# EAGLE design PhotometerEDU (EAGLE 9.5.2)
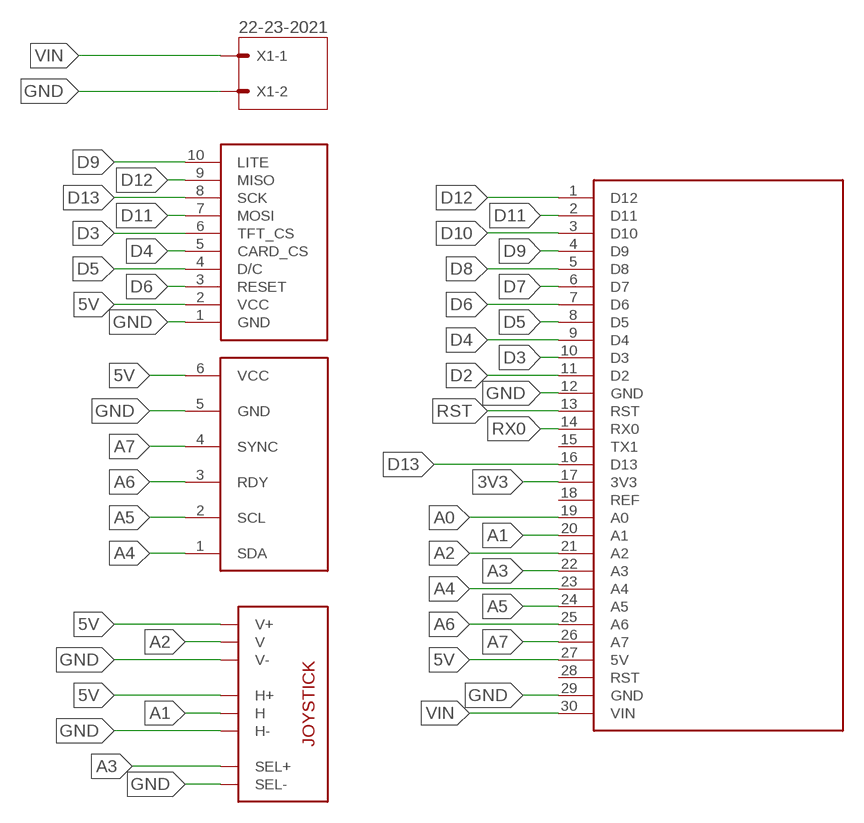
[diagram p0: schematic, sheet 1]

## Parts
78511-406  SAURON  [SAURON]
A000005  NANO  [NANO]
COM-09032  JOYSTICKPTH  [JOYSTICK]
EXP-R15-111  DISPLAY  [DISPLAY]
X1  22-23-2021  [22-23-2021]

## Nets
3V3: A000005.17(3V3)
5V: 78511-406.6(VCC) A000005.27(5V) COM-09032.H1(H+) COM-09032.V1(V+) EXP-R15-111.2(VCC)
A0: A000005.19(A0)
A1: A000005.20(A1) COM-09032.H2(H)
A2: A000005.21(A2) COM-09032.V2(V)
A3: A000005.22(A3) COM-09032.B1A(SEL+)
A4: 78511-406.1(SDA) A000005.23(A4)
A5: 78511-406.2(SCL) A000005.24(A5)
A6: 78511-406.3(RDY) A000005.25(A6)
A7: 78511-406.4(SYNC) A000005.26(A7)
D2: A000005.11(D2)
D3: A000005.10(D3) EXP-R15-111.6(TFT_CS)
D4: A000005.9(D4) EXP-R15-111.5(CARD_CS)
D5: A000005.8(D5) EXP-R15-111.4(D/C)
D6: A000005.7(D6) EXP-R15-111.3(RESET)
D7: A000005.6(D7)
D8: A000005.5(D8)
D9: A000005.4(D9) EXP-R15-111.10(LITE)
D10: A000005.3(D10)
D11: A000005.2(D11) EXP-R15-111.7(MOSI)
D12: A000005.1(D12) EXP-R15-111.9(MISO)
D13: A000005.16(D13) EXP-R15-111.8(SCK)
GND: 78511-406.5(GND) A000005.12(GND) A000005.29(GND) COM-09032.B2A(SEL-) COM-09032.H3(H-) COM-09032.V3(V-) EXP-R15-111.1(GND) X1.2
RST: A000005.13(RST)
RX0: A000005.14(RX0)
VIN: A000005.30(VIN) X1.1
Unconnected: A000005.15(TX1) A000005.18(REF) A000005.28(RST)

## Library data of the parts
78511-406 = Lego:SAURON
A000005 = Lego:NANO
COM-09032 = SparkFun-Electromechanical:JOYSTICK: Thumb Joystick Joystick commonly found in PS2 controllers. Two pots and a select switch. Footprint proven. Spark Fun Electronics SKU : COM-09032
EXP-R15-111 = Lego:DISPLAY
X1 = con-molex:22-23-2021: .100" (2.54mm) Center Header - 2 Pin; MF: MOLEX; MPN: 22-23-2021; OC_FARNELL: 1462926; OC_NEWARK: 25C3832

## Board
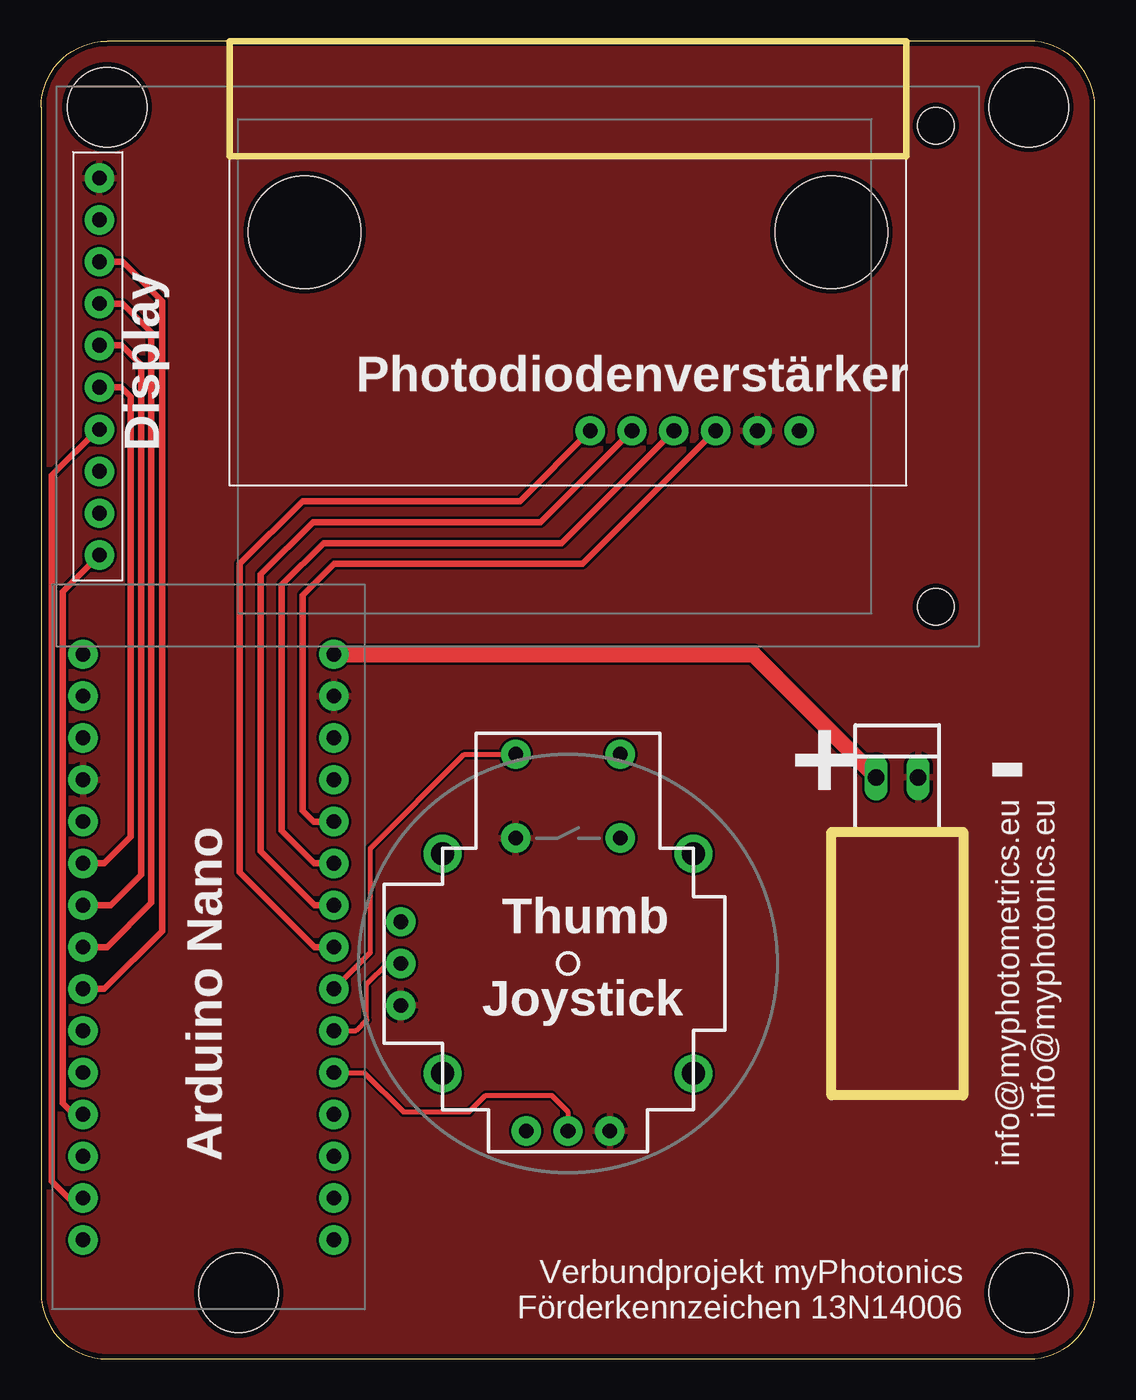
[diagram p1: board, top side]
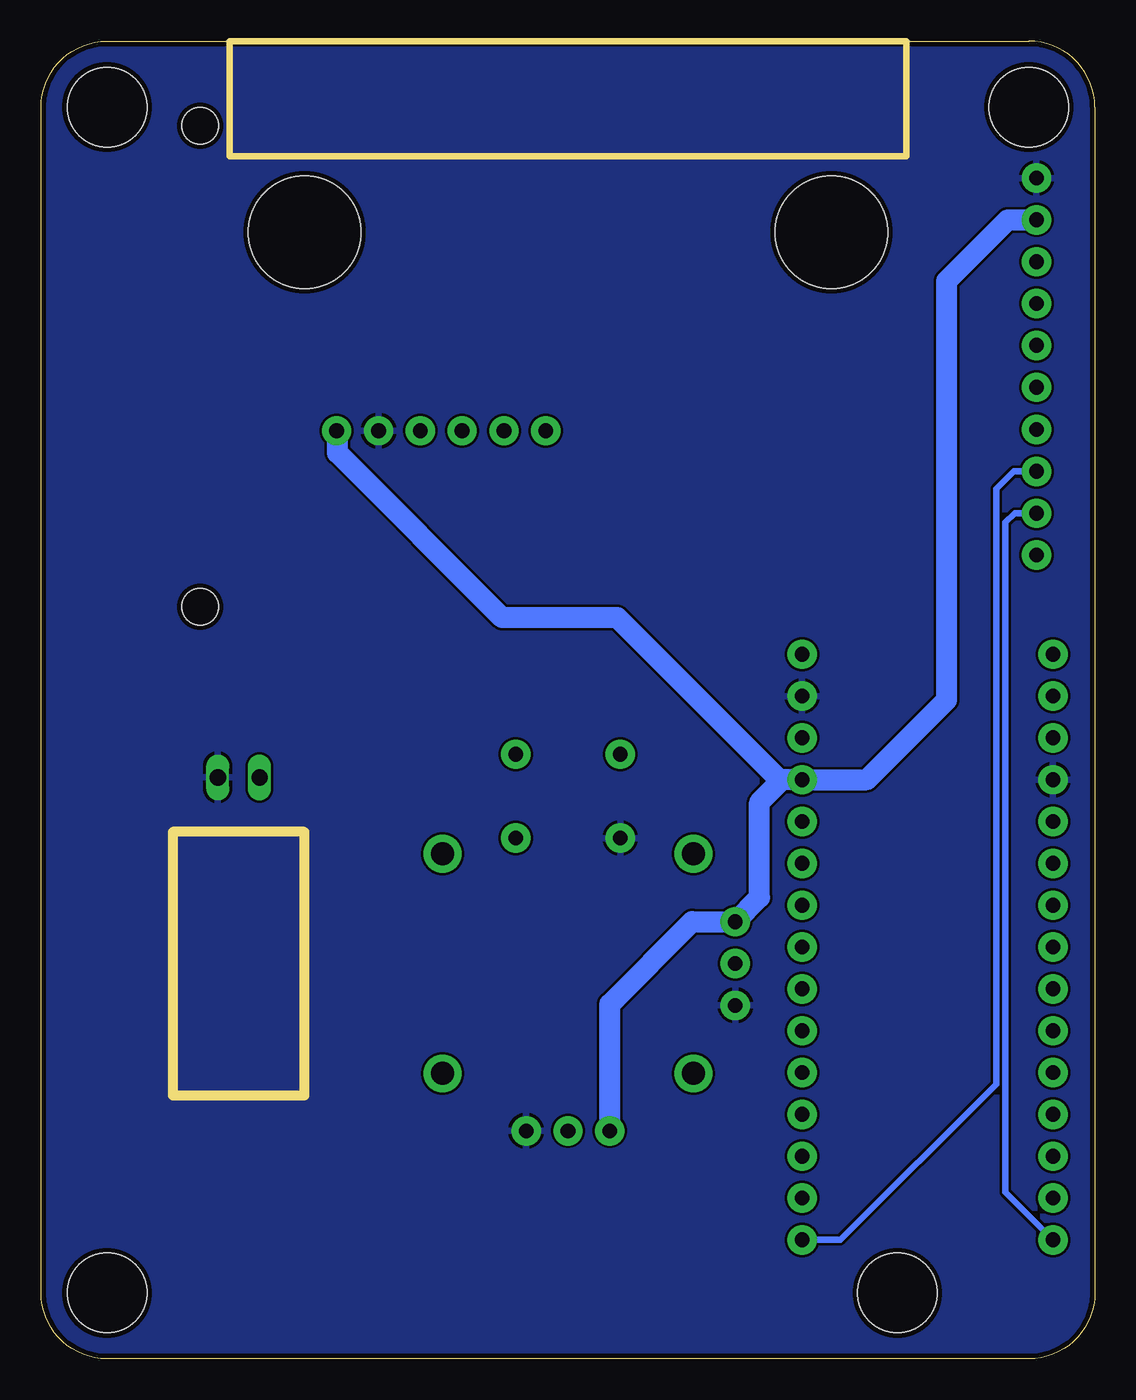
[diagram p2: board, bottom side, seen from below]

Size 64 x 80 mm. Coordinates in mm from the lower left corner, seen from the top.
Outline: 4,0 60,0 arc90 64,4 64,76 arc90 60,80 4,80 arc90 0,76 0,4 arc90 4,0
Copper layers (1*16): Top 0.035mm / dielectric 1.5mm / Bottom 0.035mm
Design rules "PCB-POOL Standard": minimum track width 0.15mm, minimum drill 0.3mm, track to track 0.15mm, track to pad 0.15mm, pad to pad 0.15mm, via to via 0.15mm, smd to smd 0.15mm, copper to edge 0.3mm, drill to drill 0.2mm, minimum pad ring 0.2mm, minimum via ring 0.15mm, stop-mask expansion 0.075mm, vias tented up to drill 0mil, thermal gap 0.2mm
Holes 4.81 mm at 60,76 60,4 12,4 4,76
Milling: area 11.4,73 to 52.6,80; area 48,16 to 56,32

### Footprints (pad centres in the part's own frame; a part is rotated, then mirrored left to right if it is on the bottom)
SAURON = drill 0.9 pad 1.778: 1 1.349,3.334; 2 3.889,3.334; 3 6.429,3.334; 4 8.969,3.334; 5 11.509,3.334; 6 14.049,3.334 | hole 6.812: -16,15.393; 16,15.393
NANO = drill 0.9 pad 1.778: 1 -17.78,7.62; 2 -15.24,7.62; 3 -12.7,7.62; 4 -10.16,7.62; 5 -7.62,7.62; 6 -5.08,7.62; 7 -2.54,7.62; 8 0,7.62; 9 2.54,7.62; 10 5.08,7.62; 11 7.62,7.62; 12 10.16,7.62; 13 12.7,7.62; 14 15.24,7.62; 15 17.78,7.62; 16 -17.78,-7.62; 17 -15.24,-7.62; 18 -12.7,-7.62; 19 -10.16,-7.62; 20 -7.62,-7.62; 21 -5.08,-7.62; 22 -2.54,-7.62; 23 0,-7.62; 24 2.54,-7.62; 25 5.08,-7.62; 26 7.62,-7.62; 27 10.16,-7.62; 28 12.7,-7.62; 29 15.24,-7.62; 30 17.78,-7.62
JOYSTICK = drill 0.9 pad 1.778: B1A -3.175,12.7; B1B 3.175,12.7; B2A -3.175,7.62; B2B 3.175,7.62 | drill 0.889 pad 1.778: H1 -2.54,-10.16; H2 0,-10.16; H3 2.54,-10.16; V1 -10.16,2.54; V2 -10.16,0; V3 -10.16,-2.54 | drill 1.397 pad 2.286: MOUNT1 -7.62,6.668; MOUNT2 -7.62,-6.668; MOUNT3 7.62,-6.668; MOUNT4 7.62,6.668
DISPLAY = drill 0.9 pad 1.778: 1 -28.46,27.94; 2 -28.46,25.4; 3 -28.46,22.86; 4 -28.46,20.32; 5 -28.46,17.78; 6 -28.46,15.24; 7 -28.46,12.67; 8 -28.46,10.13; 9 -28.46,7.59; 10 -28.46,5.05 | hole 2.2: 22.34,1.905; 22.34,31.115
22-23-2021 = drill 1 long: 1 -1.27,0; 2 1.27,0

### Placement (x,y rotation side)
78511-406  32,53.01 0 top
A000005  10.16,25 90 top
COM-09032  32,24 0 top
EXP-R15-111  32,43.75 0 top
X1  52,35.3 0 top

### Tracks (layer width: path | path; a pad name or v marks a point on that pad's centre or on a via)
5V
  Bottom 1.27: 19,35.16 A000005.27 13.84,35.16 9,40 9,65.45 5.3,69.15 EXP-R15-111.2 | 19,35.16 19.16,35.16 29,45 36,45 46,55 46,56.3 78511-406.6 | COM-09032.H1 29.46,21.54 24.46,26.54 COM-09032.V1 20.37,28.01 20.37,33.79 19,35.16
A1
  Top 0.305: A000005.20 19.62,17.38 22,15 26,15 27,16 31,16 32,15 COM-09032.H2
A2
  Top 0.305: A000005.21 19.12,19.92 19.78,20.58 19.78,22.78 21,24 COM-09032.V2
A3
  Top 0.305: A000005.22 20,24.68 20,31 25.7,36.7 COM-09032.B1A
A4
  Top 0.406: A000005.23 16.62,25 12.06,29.55 12.06,48.26 15.88,52.07 29.07,52.07 78511-406.1
A5
  Top 0.406: A000005.24 16.62,27.54 13.34,30.82 13.34,47.62 16.51,50.8 30.34,50.8 78511-406.2
A6
  Top 0.406: A000005.25 16.59,30.08 14.61,32.06 14.61,46.99 17.14,49.53 31.61,49.53 78511-406.3
A7
  Top 0.406: A000005.26 16.54,32.62 15.88,33.28 15.88,46.35 17.78,48.26 32.88,48.26 78511-406.4
D3
  Top 0.406: A000005.10 3.82,30.08 5.43,31.69 5.43,58.42 4.86,58.99 EXP-R15-111.6
D4
  Top 0.406: A000005.9 4.23,27.54 6.07,29.38 6.07,60.34 4.88,61.53 EXP-R15-111.5
D5
  Top 0.406: A000005.8 4,25 6.68,27.68 6.68,62.33 4.94,64.07 EXP-R15-111.4
D6
  Top 0.406: A000005.7 3.83,22.46 7.34,25.97 7.34,64.22 4.95,66.61 EXP-R15-111.3
D9
  Top 0.406: A000005.4 1.97,14.84 1.3,15.52 1.3,46.56 EXP-R15-111.10
D11
  Top 0.406: A000005.2 1.67,9.76 0.65,10.78 0.65,53.65 3.42,56.42 EXP-R15-111.7
D12
  Bottom 0.406: EXP-R15-111.9 4.87,51.34 5.43,50.78 5.43,10.11 A000005.1
D13
  Bottom 0.406: A000005.16 15.45,7.22 5.99,16.68 5.99,52.81 4.92,53.88 EXP-R15-111.8
GND
  pour Top: 0,0 0,80 64,80 64,0
  pour Bottom (rank 2): 0,0 0,80 64,80 64,0
VIN
  Top 1.016: A000005.30 43.25,42.78 X1.1

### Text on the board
tNames: Display | Photodiodenverstärker | + | - | info@myphotometrics.eu / info@myphotonics.eu | Thumb | Joystick | Arduino Nano | Verbundprojekt myPhotonics / Förderkennzeichen 13N14006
